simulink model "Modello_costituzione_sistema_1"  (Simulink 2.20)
settings: Solver=VariableStepDiscrete  StartTime=0.0  StopTime=10.0  RelTol=1e-3  AbsTol=1e-6
undefined symbols (not defined in the file or in its folder): Kp

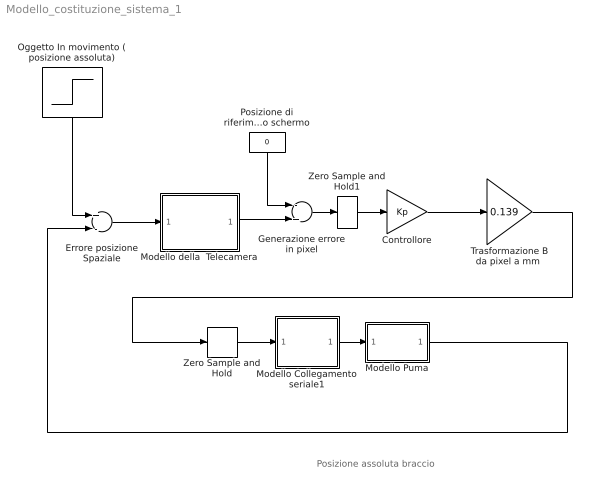
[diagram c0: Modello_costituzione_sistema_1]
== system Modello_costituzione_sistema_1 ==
  note: Posizione assoluta braccio
  Controllore : Gain  Gain=Kp
  Errore posizione Spaziale : Sum  Inputs=+-
  Generazione errore in pixel : Sum  Inputs=-+
  Modello Collegamento seriale1 : Subsystem  Description=Modello seriale
  Modello Puma : Subsystem  Description=Modello Puma
  Modello della  Telecamera : Subsystem
  Oggetto In movimento ( posizione assoluta) : Step  Orientation=down  Time=.010  Before=0  After=48.5
  Posizione di riferimento  nello schermo : Constant  Orientation=down  Value=0
  "Trasformazione B da pixel a mm " : Gain  Gain=0.139
  Zero Sample and Hold : ZeroOrderHold  SampleTime=.250
  Zero Sample and Hold1 : ZeroOrderHold  SampleTime=.070
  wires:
  Posizione di riferimento  nello schermo/1 -> Generazione errore in pixel/1
  Controllore/1 -> "Trasformazione B da pixel a mm "/1
  Modello della  Telecamera/1(Out1) -> Generazione errore in pixel/2
  Errore posizione Spaziale/1 -> Modello della  Telecamera/1(In1)
  Oggetto In movimento ( posizione assoluta)/1 -> Errore posizione Spaziale/1
  Modello Puma/1(Out1) -> Errore posizione Spaziale/2
  Zero Sample and Hold/1 -> Modello Collegamento seriale1/1(In1)
  Modello Collegamento seriale1/1(Out1) -> Modello Puma/1(In1)
  "Trasformazione B da pixel a mm "/1 -> Zero Sample and Hold/1
  Generazione errore in pixel/1 -> Zero Sample and Hold1/1
  Zero Sample and Hold1/1 -> Controllore/1

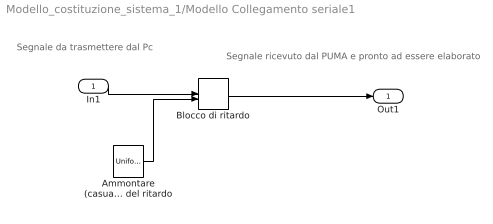
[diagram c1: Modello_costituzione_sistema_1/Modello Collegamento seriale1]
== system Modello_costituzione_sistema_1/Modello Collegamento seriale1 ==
  note: Segnale da trasmettere dal Pc
  note: Segnale ricevuto dal PUMA e pronto ad essere elaborato
  In1 : Inport  Port=1  PortWidth=-1  SampleTime=-1
  Ammontare (casuale)  in ms del ritardo : UniformRandomNumber  Minimum=.260  Maximum=.290  Seed=0  SampleTime=.280
  Blocco di ritardo : VariableTransportDelay  MaximumDelay=1  InitialInput=0  MaximumPoints=1024
  Out1 : Outport  Port=1
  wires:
  Ammontare (casuale)  in ms del ritardo/1 -> Blocco di ritardo/2
  In1/1 -> Blocco di ritardo/1
  Blocco di ritardo/1 -> Out1/1

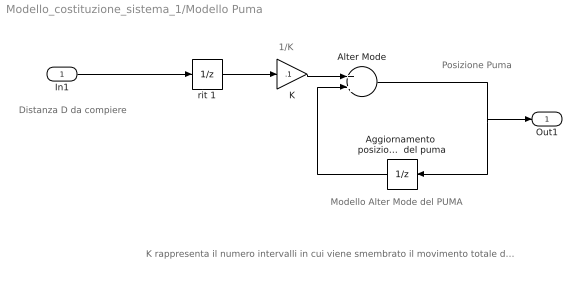
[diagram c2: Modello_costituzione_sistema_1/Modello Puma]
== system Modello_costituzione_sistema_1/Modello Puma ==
  note: Posizione Puma
  note: Modello Alter Mode del PUMA
  note: 1/K
  note: K rappresenta il numero intervalli in cui viene smembrato il movimento totale da compiere, dopo K time-slice (del PUMA) si ottiene che si e' compiuto proprio la distanza D trasmessa.
  note: Distanza D da compiere
  In1 : Inport  Port=1  PortWidth=-1  SampleTime=-1
  Aggiornamento  posizione   Il sample-time di questo blocco rappresenta la TIME-SLICE  del puma : UnitDelay  Orientation=left  X0=0  SampleTime=.034
  Alter Mode : Sum  Inputs=++
  K : Gain  Gain=.1
  rit 1 : UnitDelay  X0=0  SampleTime=.034
  Out1 : Outport  Port=1
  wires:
  Alter Mode/1 -> Aggiornamento  posizione   Il sample-time di questo blocco rappresenta la TIME-SLICE  del puma/1, Out1/1
  K/1 -> Alter Mode/1
  Aggiornamento  posizione   Il sample-time di questo blocco rappresenta la TIME-SLICE  del puma/1 -> Alter Mode/2
  rit 1/1 -> K/1
  In1/1 -> rit 1/1

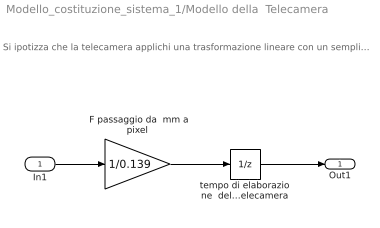
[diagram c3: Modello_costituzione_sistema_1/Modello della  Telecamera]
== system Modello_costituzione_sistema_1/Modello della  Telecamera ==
  note: Si ipotizza che la telecamera applichi una trasformazione lineare con un semplice fattore di scala F. ( ricavato automaticamente dalla procedura di calibrazione)
  In1 : Inport  Port=1  PortWidth=-1  SampleTime=-1
  " F passaggio da  mm a pixel" : Gain  Gain=1/0.139
  tempo di elaborazione  della telecamera : UnitDelay  X0=0  SampleTime=.033
  Out1 : Outport  Port=1
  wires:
  In1/1 -> " F passaggio da  mm a pixel"/1
  " F passaggio da  mm a pixel"/1 -> tempo di elaborazione  della telecamera/1
  tempo di elaborazione  della telecamera/1 -> Out1/1
